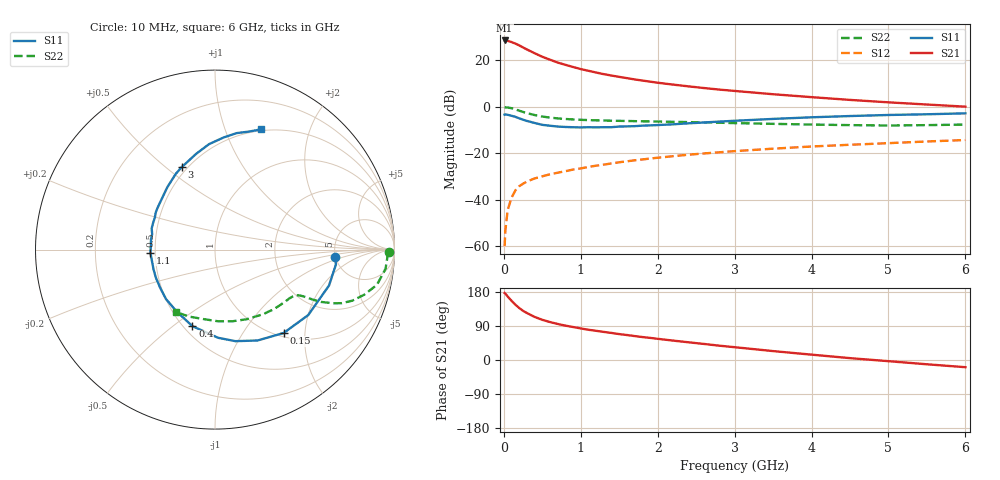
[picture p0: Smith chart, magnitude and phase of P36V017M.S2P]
! SIEMENS Small Signal Semiconductors
! BFP181
! Si NPN RF Bipolar Junction Transistor in SOT143
! VCE = 6 V  IC = 17 mA
! Common Emitter S-Parameters:  March  1996
# GHz  S  MA  R  50
!  f  S11  S21  S12  S22
! GHz  MAG  ANG  MAG  ANG  MAG  ANG  MAG  ANG
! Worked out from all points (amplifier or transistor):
!   36 points, 10 MHz to 6 GHz, reference 50 ohm
!   highest |S21| = 28.4 dB at 10 MHz (marker M1)
!   |S21| within 3 dB of that: start of sweep to 248.5 MHz
!   unconditionally stable (mu >= 1): 925.7 MHz to 5.925 GHz
!   at 250 MHz: K = 0.43, MSG = 29.3 dB, |S12| = -33.2 dB
!   at 1.4 GHz: K = 1.14, MAG = 16.7 dB, |S12| = -24.4 dB
!   at 6 GHz: K = 0.99, MSG = 7.2 dB, |S12| = -14.4 dB
!   S11 on the Smith chart (normalised r, x): 10 MHz: 4.97, -0.74; 150 MHz: 1.07, -1.56; 400 MHz: 0.55, -0.59; 1.1 GHz: 0.47, -0.02; 3 GHz: 0.47, +0.57; 6 GHz: 0.49, +1.33
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0.01  0.6711 -3.5  26.39 176.7  0.001 76.4  0.969 -0.9
0.02  0.6789 -7.0  26.27 175.0  0.0022 83.0  0.9619 -2.3
0.05  0.666 -17.5  25.88 167.6  0.006 84.3  0.9563 -6.4
0.1  0.6346 -35.1  24.36 156.2  0.011 73.2  0.9233 -12.3
0.15  0.6018 -50.5  22.58 146.0  0.0158 68.4  0.8687 -16.8
0.2  0.5591 -64.9  20.67 137.2  0.0194 63.1  0.8161 -20.4
0.25  0.5228 -77.4  18.62 129.7  0.022 60.8  0.7669 -22.9
0.3  0.4916 -88.0  16.92 124.0  0.0245 58.0  0.7239 -24.4
0.4  0.4449 -106.4  14.01 113.7  0.0286 55.5  0.6577 -26.3
0.5  0.4055 -121.9  11.76 106.0  0.0317 53.0  0.6116 -27.1
0.6  0.3879 -134.7  10.19 100.1  0.0351 53.5  0.5794 -27.5
0.7  0.3722 -145.2  8.829 95.1  0.0379 53.7  0.5573 -27.9
0.9  0.3598 -162.2  7.101 87.0  0.0443 53.3  0.5293 -28.8
1.1  0.3602 -177.3  5.878 79.8  0.0505 53.7  0.5124 -30.1
1.5  0.372 161.6  4.353 68.4  0.0636 53.7  0.4939 -33.8
1.8  0.3894 148.0  3.629 60.6  0.073 52.5  0.4825 -37.7
2.2  0.4158 134.0  2.969 51.2  0.0859 50.3  0.4701 -43.3
3  0.4953 112.0  2.17 33.8  0.1103 44.5  0.4413 -56.3
3.5  0.5435 101.2  1.843 23.5  0.1246 40.7  0.4258 -65.8
4.5  0.6265 85.6  1.392 4.9  0.1512 32.6  0.3996 -87.6
5.5  0.6839 74.0  1.108 -11.3  0.1779 25.3  0.3995 -110.6
6  0.7161 69.2  0.997 -19.0  0.191 20.9  0.411 -122.3
